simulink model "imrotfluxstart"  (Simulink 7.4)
settings: Solver=ode45  StartTime=0.0  StopTime=2  MaxStep=1e-4  RelTol=1e-3  AbsTol=1e-3

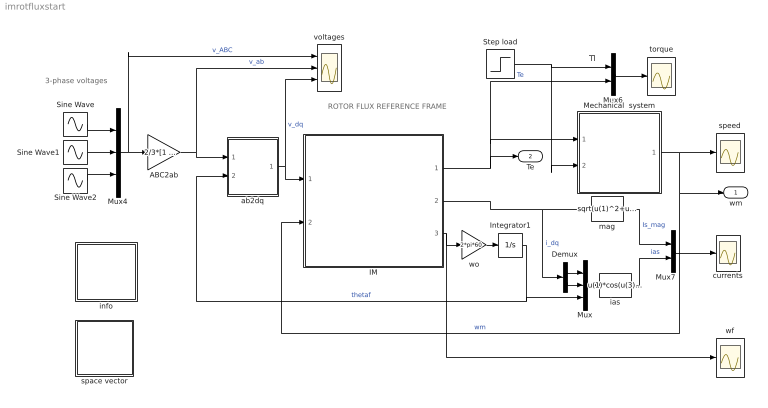
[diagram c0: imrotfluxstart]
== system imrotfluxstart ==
  note: ROTOR FLUX REFERENCE FRAME
  note: Tl
  note: 3-phase voltages
  ABC2ab : Gain  Gain=2/3*[1 -0.5 -0.5;0 sqrt(3)/2 -sqrt(3)/2]  Multiplication=Matrix(K*u)  ParameterDataType=sfix(16)  ParameterScaling=2^0  OutDataType=sfix(16)  OutScaling=2^0
  Demux : Demux  Outputs=2
  IM : Subsystem  mask{Rs=0.01, Rr=0.02, Lsl=0.10, Lrl=0.10, Lm=4.50, wo=2*pi*60}
      mask prompts: Rs "Stator resistance [pu]"; Rr "Rotor resistance [pu]"; Lsl "Stator leakage inductance [pu]"; Lrl "Rotor leakage inductance [pu]"; Lm "Magnetizing inductance [pu]"; wo "Base frequency"
  Integrator1 : Integrator
  Mechanical  system : Subsystem  mask{H=0.30, Bm=1e-5}
      mask prompts: H "Inertia constant [s]"; Bm "Damping coefficient [pu]"
  Mux : Mux  Inputs=3
  Mux4 : Mux  Inputs=3
  Mux6 : Mux  Inputs=2
  Mux7 : Mux  Inputs=2
  Sine Wave : Sin  Amplitude=1  Bias=0  Frequency=2*pi*60  Phase=pi  Samples=10  SampleTime=0
  Sine Wave1 : Sin  Amplitude=1  Bias=0  Frequency=2*pi*60  Phase=pi-2*pi/3  Samples=10  SampleTime=0
  Sine Wave2 : Sin  Amplitude=1  Bias=0  Frequency=2*pi*60  Phase=pi+2*pi/3  Samples=10  SampleTime=0
  Step load : Step  Time=1.5  Before=0.0  SampleTime=0
  ab2dq : Subsystem
  currents : Scope
  ias : Fcn  Expr=u(1)*cos(u(3))-u(2)*sin(u(3))
  info : Subsystem
  mag : Fcn  Expr=sqrt(u(1)^2+u(2)^2)
  space vector : Subsystem
  speed : Scope
  torque : Scope
  voltages : Scope  NumInputPorts=3
  wf : Scope
  wo : Gain  Gain=2*pi*60  ParameterDataType=sfix(16)  ParameterScaling=2^0  OutDataType=sfix(16)  OutScaling=2^0
  wm : Outport
  Te : Outport  Port=2
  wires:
  Mux6/1 -> torque/1
  Mechanical  system/1(wm) -> speed/1, IM/2(wm), wm/1  "wm"
  ab2dq/1(dq) -> IM/1(vs), voltages/3  "v_dq"
  Mux4/1 -> ABC2ab/1, voltages/1  "v_ABC"
  ABC2ab/1 -> ab2dq/1(ab), voltages/2  "v_ab"
  Sine Wave/1 -> Mux4/1
  Sine Wave1/1 -> Mux4/2
  Sine Wave2/1 -> Mux4/3
  Step load/1 -> Mux6/1, Mechanical  system/2(Tl)
  Demux/1 -> Mux/1
  Demux/2 -> Mux/2
  Mux/1 -> ias/1
  ias/1 -> Mux7/2  "ias"
  mag/1 -> Mux7/1  "Is_mag"
  Mux7/1 -> currents/1
  IM/2(is) -> mag/1, Demux/1  "i_dq"
  IM/1(Te) -> Te/1, Mux6/2, Mechanical  system/1(Te)  "Te"
  wo/1 -> Integrator1/1
  IM/3(wf) -> wo/1, wf/1
  Integrator1/1 -> Mux/3, ab2dq/2(thetak)  "thetaf"

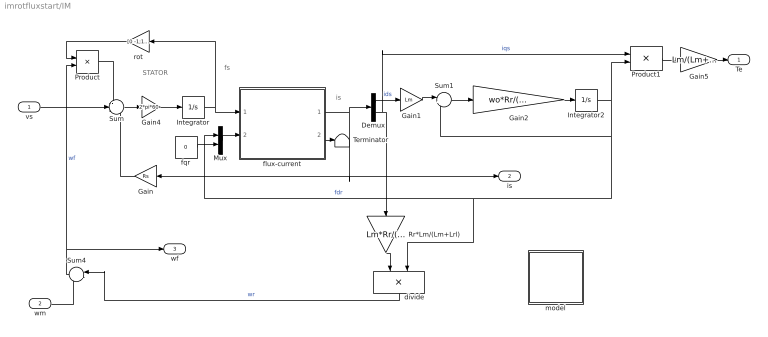
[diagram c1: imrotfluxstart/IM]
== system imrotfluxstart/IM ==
  note: STATOR
  note: fs
  note: is
  vs : Inport  OutDataType=sfix(16)  OutScaling=2^0
  wm : Inport  Port=2  OutDataType=sfix(16)  OutScaling=2^0
  Demux : Demux  Outputs=2
  Gain : Gain  Gain=Rs  ParameterDataType=sfix(16)  ParameterScaling=2^0  OutDataType=sfix(16)  OutScaling=2^0
  Gain1 : Gain  Gain=Lm  ParameterDataType=sfix(16)  ParameterScaling=2^0  OutDataType=sfix(16)  OutScaling=2^0
  Gain2 : Gain  Gain=wo*Rr/(Lm+Lrl)  ParameterDataType=sfix(16)  ParameterScaling=2^0  OutDataType=sfix(16)  OutScaling=2^0
  Gain4 : Gain  Gain=2*pi*60  ParameterDataType=sfix(16)  ParameterScaling=2^0  OutDataType=sfix(16)  OutScaling=2^0
  Gain5 : Gain  Gain=Lm/(Lm+Lrl)  ParameterDataType=sfix(16)  ParameterScaling=2^0  OutDataType=sfix(16)  OutScaling=2^0
  Integrator : Integrator  InitialCondition=[0 0]
  Integrator2 : Integrator  InitialCondition=1e-5
  Mux : Mux  Inputs=2
  Product : Product  OutDataType=sfix(16)  OutScaling=2^0
  Product1 : Product  OutDataType=sfix(16)  OutScaling=2^0
  Rr*Lm/(Lm+Lrl) : Gain  Gain=Lm*Rr/(Lm+Lrl)  ParameterDataType=sfix(16)  ParameterScaling=2^0  OutDataType=sfix(16)  OutScaling=2^0
  Sum : Sum  Inputs=-+-  OutDataType=sfix(16)  OutScaling=2^0
  Sum1 : Sum  Inputs=|+-  OutDataType=sfix(16)  OutScaling=2^0
  Sum4 : Sum  Inputs=|++  OutDataType=sfix(16)  OutScaling=2^0
  Terminator : Terminator
  divide : Product  Inputs=*/  OutDataType=sfix(16)  OutScaling=2^0
  flux-current : Subsystem
  fqr : Constant  Value=0  OutDataType=sfix(16)  OutScaling=2^0
  model : Subsystem
  rot : Gain  Gain=[0 -1;1 0]  Multiplication=Matrix(K*u)  ParameterDataType=sfix(16)  ParameterScaling=2^0  OutDataType=sfix(16)  OutScaling=2^0
  Te : Outport
  is : Outport  Port=2
  wf : Outport  Port=3
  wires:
  Gain/1 -> Sum/3
  Integrator/1 -> flux-current/1(fs), rot/1
  Product/1 -> Sum/1
  rot/1 -> Product/1
  Sum/1 -> Gain4/1
  Gain4/1 -> Integrator/1
  flux-current/1(is) -> Gain/1, is/1, Demux/1
  vs/1 -> Sum/2
  wm/1 -> Sum4/2
  Rr*Lm/(Lm+Lrl)/1 -> divide/1
  Demux/1 -> Gain1/1  "ids"
  Sum4/1 -> Product/2, wf/1  "wf"
  divide/1 -> Sum4/1  "wr"
  fqr/1 -> Mux/2
  Demux/2 -> Rr*Lm/(Lm+Lrl)/1, Product1/1  "iqs"
  Gain1/1 -> Sum1/1
  Sum1/1 -> Gain2/1
  Gain2/1 -> Integrator2/1
  Integrator2/1 -> divide/2, Mux/1, Sum1/2, Product1/2  "fdr"
  Product1/1 -> Gain5/1
  Gain5/1 -> Te/1
  Mux/1 -> flux-current/2(fr)
  flux-current/2(ir) -> Terminator/1

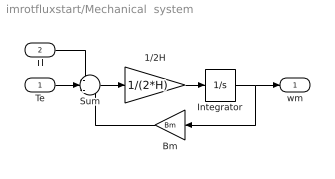
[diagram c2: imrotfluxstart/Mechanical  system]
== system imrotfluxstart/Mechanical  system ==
  Te : Inport  OutDataType=sfix(16)  OutScaling=2^0
  Tl : Inport  Port=2  OutDataType=sfix(16)  OutScaling=2^0
  1/2H : Gain  Gain=1/(2*H)  ParameterDataType=sfix(16)  ParameterScaling=2^0  OutDataType=sfix(16)  OutScaling=2^0
  Bm : Gain  Gain=Bm  ParameterDataType=sfix(16)  ParameterScaling=2^0  OutDataType=sfix(16)  OutScaling=2^0
  Integrator : Integrator
  Sum : Sum  Inputs=-+-  OutDataType=sfix(16)  OutScaling=2^0
  wm : Outport
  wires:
  1/2H/1 -> Integrator/1
  Sum/1 -> 1/2H/1
  Bm/1 -> Sum/3
  Integrator/1 -> Bm/1, wm/1
  Te/1 -> Sum/2
  Tl/1 -> Sum/1

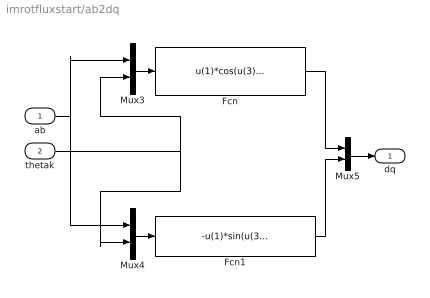
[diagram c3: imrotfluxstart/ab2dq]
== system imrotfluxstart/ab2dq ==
  ab : Inport  OutDataType=sfix(16)  OutScaling=2^0
  thetak : Inport  Port=2  OutDataType=sfix(16)  OutScaling=2^0
  Fcn : Fcn  Expr=u(1)*cos(u(3))+u(2)*sin(u(3))
  Fcn1 : Fcn  Expr=-u(1)*sin(u(3))+u(2)*cos(u(3))
  Mux3 : Mux  Inputs=2
  Mux4 : Mux  Inputs=2
  Mux5 : Mux  Inputs=2
  dq : Outport
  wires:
  Mux3/1 -> Fcn/1
  Mux4/1 -> Fcn1/1
  ab/1 -> Mux3/1, Mux4/1
  thetak/1 -> Mux3/2, Mux4/2
  Fcn1/1 -> Mux5/2
  Fcn/1 -> Mux5/1
  Mux5/1 -> dq/1

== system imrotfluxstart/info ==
  note: Line Start of an Induction Motor Modeled in the Rotor Flux Frame under Three-Phase Sinusoidal Excitation

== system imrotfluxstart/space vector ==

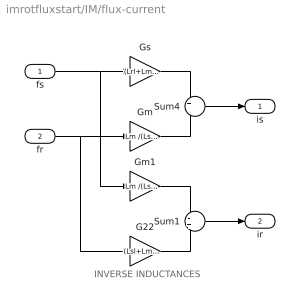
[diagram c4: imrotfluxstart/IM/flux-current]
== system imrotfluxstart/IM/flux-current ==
  note: INVERSE INDUCTANCES
  fs : Inport  OutDataType=sfix(16)  OutScaling=2^0
  fr : Inport  Port=2  OutDataType=sfix(16)  OutScaling=2^0
  G22 : Gain  Gain=(Lsl+Lm )/(Lsl*Lrl+Lsl*Lm+Lrl*Lm)  ParameterDataType=sfix(16)  ParameterScaling=2^0  OutDataType=sfix(16)  OutScaling=2^0
  Gm : Gain  Gain=Lm /(Lsl*Lrl+Lsl*Lm+Lrl*Lm)  ParameterDataType=sfix(16)  ParameterScaling=2^0  OutDataType=sfix(16)  OutScaling=2^0
  Gm1 : Gain  Gain=Lm /(Lsl*Lrl+Lsl*Lm+Lrl*Lm)  ParameterDataType=sfix(16)  ParameterScaling=2^0  OutDataType=sfix(16)  OutScaling=2^0
  Gs : Gain  Gain=(Lrl+Lm) /(Lsl*Lrl+Lsl*Lm+Lrl*Lm)  ParameterDataType=sfix(16)  ParameterScaling=2^0  OutDataType=sfix(16)  OutScaling=2^0
  Sum1 : Sum  Inputs=-+  OutDataType=sfix(16)  OutScaling=2^0
  Sum4 : Sum  Inputs=+-  OutDataType=sfix(16)  OutScaling=2^0
  is : Outport
  ir : Outport  Port=2
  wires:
  fs/1 -> Gs/1, Gm1/1
  Gs/1 -> Sum4/1
  fr/1 -> Gm/1, G22/1
  Gm/1 -> Sum4/2
  Sum4/1 -> is/1
  Gm1/1 -> Sum1/1
  G22/1 -> Sum1/2
  Sum1/1 -> ir/1

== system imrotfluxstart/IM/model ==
  note: Mathematical model of the induction machine described in the rotor flux reference frame. (Per unit formulation)
  note: Electrical system equations: vs = Rs is + 1/wo (dfs/dt) + wf M(pi/2) fs where the variables is, vs, and fs are 2-dimensional space vectors and M(pi/2) represents a 90o space rotator namely [0 -1;1 0] wf = wm + wr; wr = Rr Lm/Lr (iqs / fdr) 1/wo Lr/Rr (dfdr/dt) + fdr = Lm ids fqr = 0 The flux linkage current relations : fs = Ls is + Lm ir fr = Lm is + Lr ir Ls= Lm + Lsl ; Lr = Lm + Lrl Mechanical system equations: Te = 2H (dwm/dt) + Bm wm + Tl where Te = Lm/Lr (iqs fdr)
